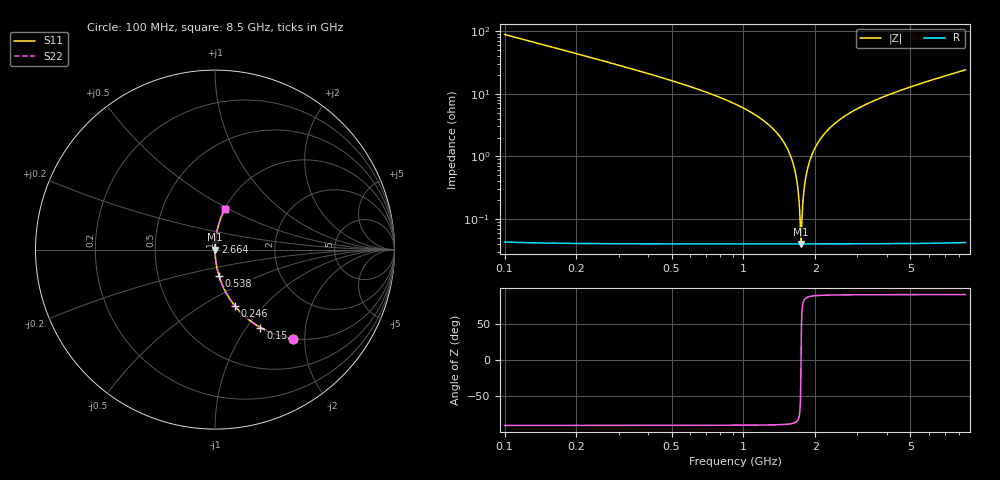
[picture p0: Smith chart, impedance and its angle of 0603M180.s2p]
! Created Wed Apr 18 16:42:31 2012
# hz S ma R 50
! 2 Port Network Data from SP1.SP block
! freq  magS11  angS11  magS21  angS21  magS12  angS12  magS22  angS22
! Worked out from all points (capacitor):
!   8401 points, 100 MHz to 8.5 GHz, reference 50 ohm
!   read as one part in series: C = 18.1 pF near 142 MHz
!   lowest |Z| = 40.6 mohm at 1.742 GHz (marker M1)
!   series resonance near 1.742 GHz, so ESL is about 460 pH
!   S11 on the Smith chart (normalised r, x): 100 MHz: 1.00, -1.75; 150 MHz: 1.00, -1.16; 246 MHz: 1.00, -0.70; 538 MHz: 1.00, -0.30; 2.664 GHz: 1.00, +0.09; 8.5 GHz: 1.00, +0.48
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1e8  0.6585 -48.8  0.7522 41.2  0.7522 41.2  0.6585 -48.8
1.5e8  0.5024 -59.8  0.8643 30.2  0.8643 30.2  0.5024 -59.8
2.46e8  0.3302 -70.7  0.9435 19.3  0.9435 19.3  0.3302 -70.7
5.38e8  0.1461 -81.4  0.9889 8.4  0.9889 8.4  0.1461 -81.4
1.208e9  0.03774 -87.2  0.9989 2.2  0.9989 2.2  0.03774 -87.2
1.5e9  0.01517 -87.6  0.9995 0.9  0.9995 0.9  0.01517 -87.6
1.581e9  0.009829 -87.1  0.9995 0.6  0.9995 0.6  0.009829 -87.1
1.64e9  0.006128 -85.9  0.9996 0.4  0.9996 0.4  0.006128 -85.9
1.679e9  0.003764 -83.6  0.9996 0.2  0.9996 0.2  0.003764 -83.6
1.717e9  0.001539 -74.7  0.9996 0.1  0.9996 0.1  0.001539 -74.7
1.742e9  0.0004054 -3.9  0.9996 0.0  0.9996 0.0  0.0004054 -3.9
1.768e9  0.001521 74.5  0.9996 -0.1  0.9996 -0.1  0.001521 74.5
1.806e9  0.003634 83.4  0.9996 -0.2  0.9996 -0.2  0.003634 83.4
1.845e9  0.005783 85.7  0.9996 -0.3  0.9996 -0.3  0.005783 85.7
1.984e9  0.01313 87.5  0.9995 -0.8  0.9995 -0.8  0.01313 87.5
2.248e9  0.02597 87.6  0.9993 -1.5  0.9993 -1.5  0.02597 87.6
2.664e9  0.0441 86.9  0.9986 -2.5  0.9986 -2.5  0.0441 86.9
2.9e9  0.0536 86.5  0.9982 -3.1  0.9982 -3.1  0.0536 86.5
4.3e9  0.1038 83.8  0.9942 -6.0  0.9942 -6.0  0.1038 83.8
5.7e9  0.1488 81.3  0.9885 -8.6  0.9885 -8.6  0.1488 81.3
7.1e9  0.1914 78.8  0.9811 -11.0  0.9811 -11.0  0.1914 78.8
8.5e9  0.2327 76.4  0.9721 -13.5  0.9721 -13.5  0.2327 76.4
